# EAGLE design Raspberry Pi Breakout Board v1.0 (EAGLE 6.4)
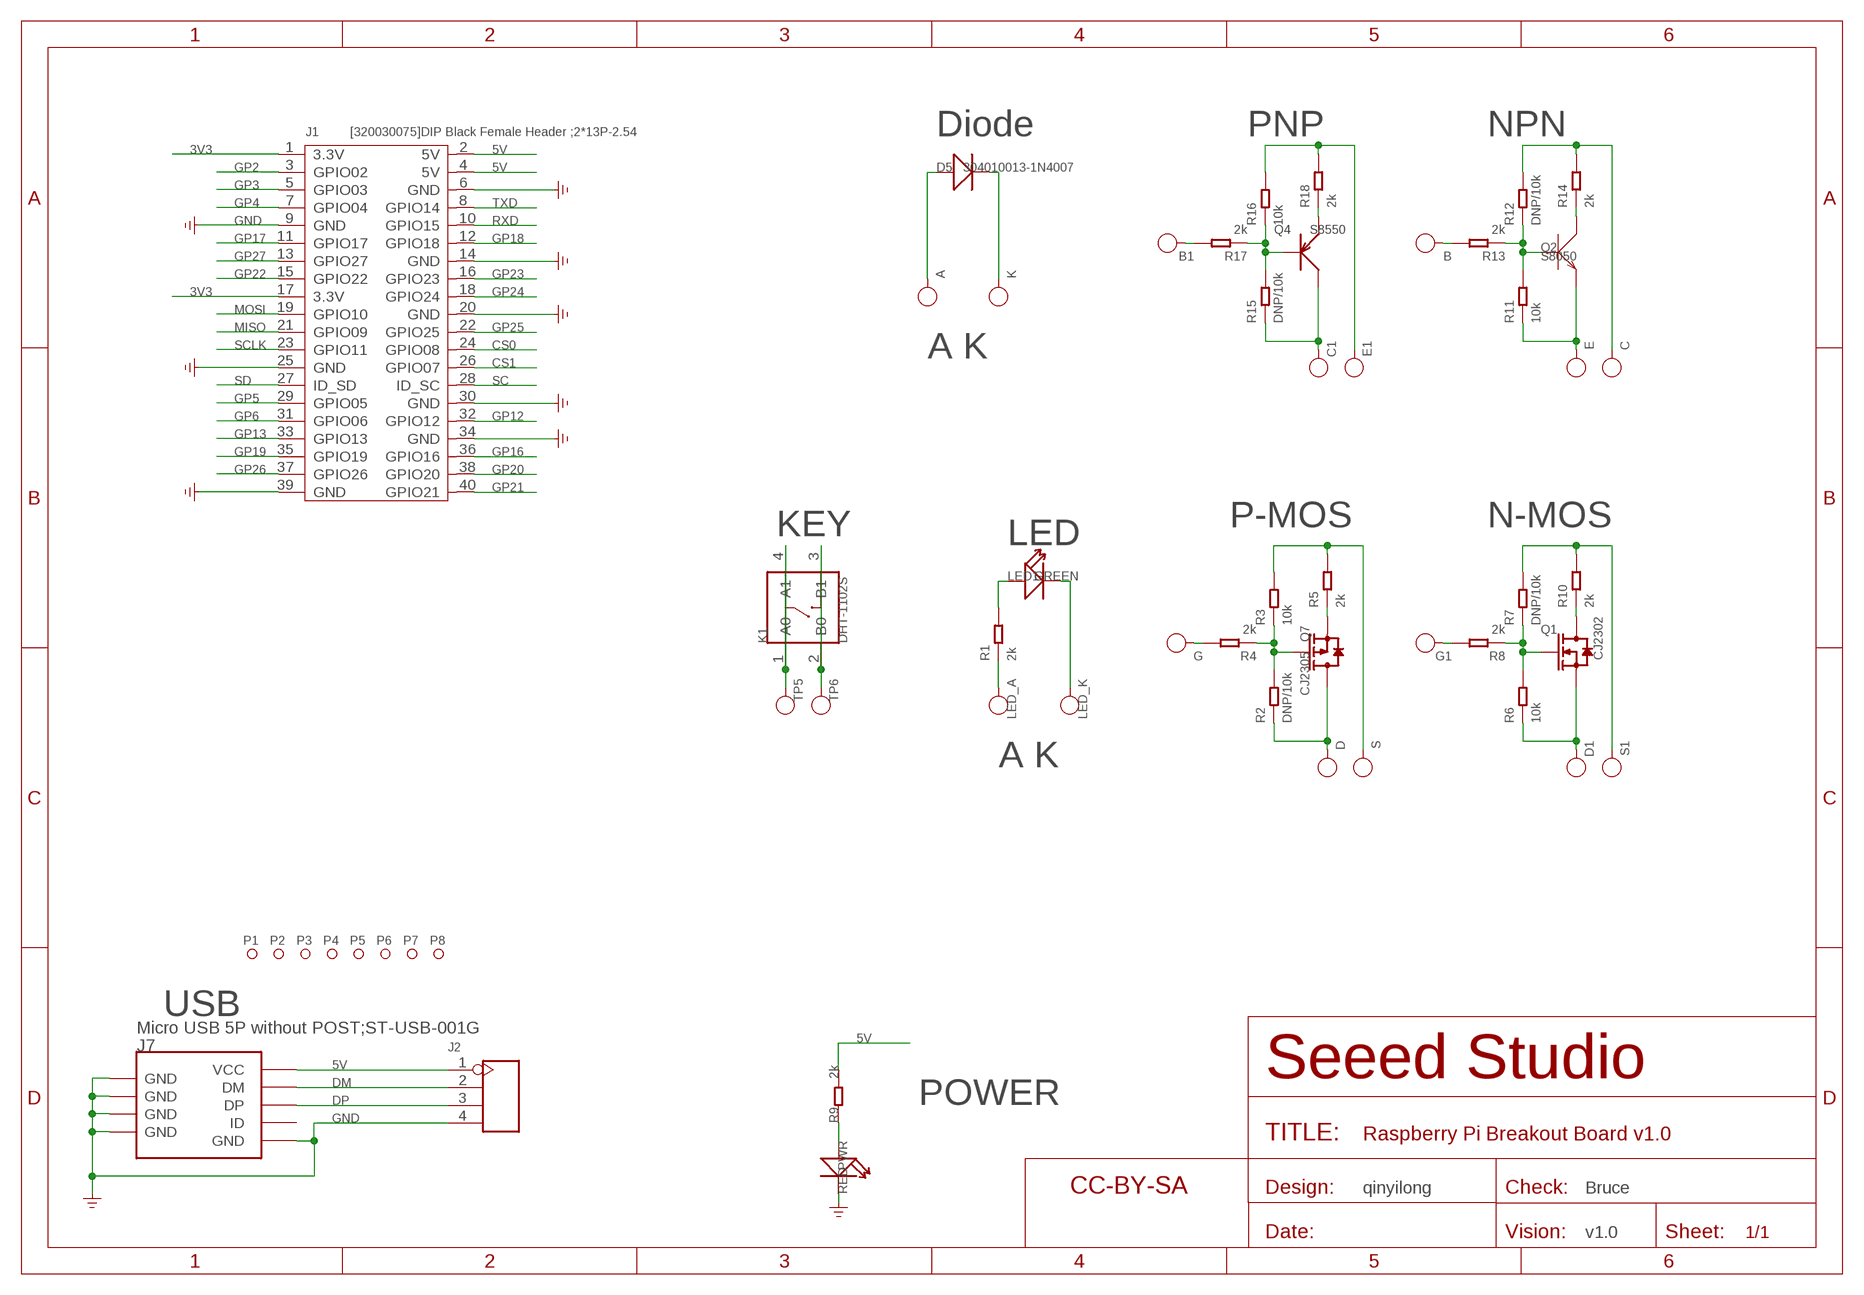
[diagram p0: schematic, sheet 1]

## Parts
A  PAD-TEST-POINT'4080'  [PAD-L80*W40MIL]
B  PAD-TEST-POINT'4080'  [PAD-L80*W40MIL]
B1  PAD-TEST-POINT'4080'  [PAD-L80*W40MIL]
C  PAD-TEST-POINT'4080'  [PAD-L80*W40MIL]
C1  PAD-TEST-POINT'4080'  [PAD-L80*W40MIL]
D  PAD-TEST-POINT'4080'  [PAD-L80*W40MIL]
D1  PAD-TEST-POINT'4080'  [PAD-L80*W40MIL]
D5  304010013-1N4007  D'DO-214AC'  [D2010]
E  PAD-TEST-POINT'4080'  [PAD-L80*W40MIL]
E1  PAD-TEST-POINT'4080'  [PAD-L80*W40MIL]
G  PAD-TEST-POINT'4080'  [PAD-L80*W40MIL]
G1  PAD-TEST-POINT'4080'  [PAD-L80*W40MIL]
J1  [320030075]DIP Black Female Header ;2*13P-2.54  HEADER-2X20P  [2X20P-2.54-65/35MIL]
J2  HEADER-4P-65/35MIL  [4P-2.54-65/35MIL]
J7  Micro USB 5P without POST;ST-USB-001G  USB-MINIUSB-5P-MICRO  [MICRO-USB]
K  PAD-TEST-POINT'4080'  [PAD-L80*W40MIL]
K1  DHT-1102S  BUTTON-4PDTSM-62K-S-V-T/R(SN431)  [4P-SMD-L6.0*W6.0*H5.0MM]
LED1  GREEN  LED'0603'  [LED-0603]
LED_A  PAD-TEST-POINT'4080'  [PAD-L80*W40MIL]
LED_K  PAD-TEST-POINT'4080'  [PAD-L80*W40MIL]
P1  PAD-MARK'ANNULAR'  [ROUND-MARK-1.0]
P2  PAD-MARK'ANNULAR'  [ROUND-MARK-1.0]
P3  PAD-MARK'ANNULAR'  [ROUND-MARK-1.0]
P4  PAD-MARK'ANNULAR'  [ROUND-MARK-1.0]
P5  PAD-MARK'ANNULAR'  [ROUND-MARK-1.0]
P6  PAD-MARK'ANNULAR'  [ROUND-MARK-1.0]
P7  PAD-MARK'ANNULAR'  [ROUND-MARK-1.0]
P8  PAD-MARK'ANNULAR'  [ROUND-MARK-1.0]
PWR  RED  LED'0603'  [LED-0603]
Q1  CJ2302  MOSFET-N'SOT23'  [SOT23]
Q2  S8050  TRANSISTOR-NPN-SOT23  [SOT23]
Q4  S8550  TRANSISTOR-PNP-SOT23  [SOT23]
Q7  CJ2305  MOSFET-P'SI2323CDS/SI2305DS<BR>'  [SOT23]
R1  2k  RES-0603  [R0603]
R2  DNP/10k  RES-0603  [R0603]
R3  10k  RES-0603  [R0603]
R4  2k  RES-0603  [R0603]
R5  2k  RES-0603  [R0603]
R6  10k  RES-0603  [R0603]
R7  DNP/10k  RES-0603  [R0603]
R8  2k  RES-0603  [R0603]
R9  2k  R-0603  [R0603]
R10  2k  RES-0603  [R0603]
R11  10k  RES-0603  [R0603]
R12  DNP/10k  RES-0603  [R0603]
R13  2k  RES-0603  [R0603]
R14  2k  RES-0603  [R0603]
R15  DNP/10k  RES-0603  [R0603]
R16  10k  RES-0603  [R0603]
R17  2k  RES-0603  [R0603]
R18  2k  RES-0603  [R0603]
S  PAD-TEST-POINT'4080'  [PAD-L80*W40MIL]
S1  PAD-TEST-POINT'4080'  [PAD-L80*W40MIL]
TP5  PAD-TEST-POINT'4080'  [PAD-L80*W40MIL]
TP6  PAD-TEST-POINT'4080'  [PAD-L80*W40MIL]
U$2  SEEEDSTUDIO-OPEN-SCH-FRAME  [SEEEDSTUDIO-PCB-FRAME]

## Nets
3V3: J1.1(3.3V) J1.17(3.3V)
5V: J1.2(5V) J1.4(5V) J2.1 J7.1(VCC) R9.2
CS0: J1.24(GPIO08)
CS1: J1.26(GPIO07)
DM: J2.2 J7.2(DM)
DP: J2.3 J7.3(DP)
GND: J1.6(GND) J1.9(GND) J1.14(GND) J1.20(GND) J1.25(GND) J1.30(GND) J1.34(GND) J1.39(GND) J2.4 J7.5(GND) J7.S1(GND) J7.S2(GND) J7.S3(GND) J7.S4(GND) J7.S5(GND) J7.S6(GND) PWR.- ; supply symbol labelled GND_POWER
GP2: J1.3(GPIO02)
GP3: J1.5(GPIO03)
GP4: J1.7(GPIO04)
GP5: J1.29(GPIO05)
GP6: J1.31(GPIO06)
GP12: J1.32(GPIO12)
GP13: J1.33(GPIO13)
GP16: J1.36(GPIO16)
GP17: J1.11(GPIO17)
GP18: J1.12(GPIO18)
GP19: J1.35(GPIO19)
GP20: J1.38(GPIO20)
GP21: J1.40(GPIO21)
GP22: J1.15(GPIO22)
GP23: J1.16(GPIO23)
GP24: J1.18(GPIO24)
GP25: J1.22(GPIO25)
GP26: J1.37(GPIO26)
GP27: J1.13(GPIO27)
MISO: J1.21(GPIO09)
MOSI: J1.19(GPIO10)
N$320: LED_A.1(T) R1.1
N$336: C1.1(T) Q4.3(C) R15.1
N$347: Q7.1(G) R2.2 R3.1 R4.1
N$370: R3.2 R5.2 S.1(T)
N$373: D1.1(T) Q1.2(S) R6.1
N$374: G.1(T) R4.2
N$375: Q7.2(S) R5.1
N$376: Q1.1(G) R6.2 R7.1 R8.1
N$377: PWR.+ R9.1
N$378: Q4.1(B) R15.2 R16.1 R17.1
N$379: E1.1(T) R16.2 R18.2
N$380: B1.1(T) R17.2
N$381: Q4.2(E) R18.1
N$383: R7.2 R10.2 S1.1(T)
N$384: G1.1(T) R8.2
N$385: D.1(T) Q7.3(D) R2.1
N$386: E.1(T) Q2.2(E) R11.1
N$387: Q2.1(B) R11.2 R12.1 R13.1
N$388: C.1(T) R12.2 R14.2
N$389: A.1(T) D5.+
N$390: D5.- K.1(T)
N$391: LED1.+ R1.2
N$392: LED1.- LED_K.1(T)
N$393: K1.1(A0) K1.4(A1) TP5.1(T)
N$394: K1.2(B0) K1.3(B1) TP6.1(T)
N$395: Q1.3(D) R10.1
N$396: B.1(T) R13.2
N$397: Q2.3(C) R14.1
RXD: J1.10(GPIO15)
SC: J1.28(ID_SC)
SCLK: J1.23(GPIO11)
SD: J1.27(ID_SD)
TXD: J1.8(GPIO14)
Unconnected: J7.4(ID)

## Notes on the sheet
- Diode | PNP | NPN
- A K
- KEY | P-MOS | N-MOS
- LED
- A K
- USB
- POWER
- qinyilong | Bruce
- v1.0

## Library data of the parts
A B B1 C C1 D D1 E E1 G G1 K LED_A LED_K S S1 TP5 TP6 = Discrete-new:PAD-TEST-POINT
D5 = Discrete:D*
J1 = Connector-new:HEADER-2X20P
J2 = Connector-new:HEADER-4P
J7 = Connector :USB-MINIUSB-5P
K1 = Discrete-new:BUTTON-4P: 4P-L6.0*W6.0*H5.0mm:311020024;4P-L8.0*W8.0*H9.0MM:311020028;4P-SMD-L6.0*W6.0*H5.0MM:311020004;4P-SMD-L3.35*W3.35*H1.5MM:311020030;4P-SMD-L5.2*W5.2*H2.5:311020046
LED1 PWR = Discrete:LED*
P1-P8 = Discrete-new:PAD-MARK; PARTNO: DNP
Q1 = Discrete:MOSFET-N: IRLL014: http://www.vishay.com/docs/91319/sihll014.pdf
Q2 = Discrete:TRANSISTOR-NPN*: NPN audion
Q4 = Discrete:TRANSISTOR-PNP*: PNP audion
Q7 = Discrete:MOSFET-P
R1-R8 R10-R18 = Discrete-new:RES
R9 = Discrete:R*
U$2 = moudle-new:SEEEDSTUDIO-OPEN-SCH-FRAME

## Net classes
0 default: width 0.076 mm, drill 0.102 mm, clearance 0.076 mm

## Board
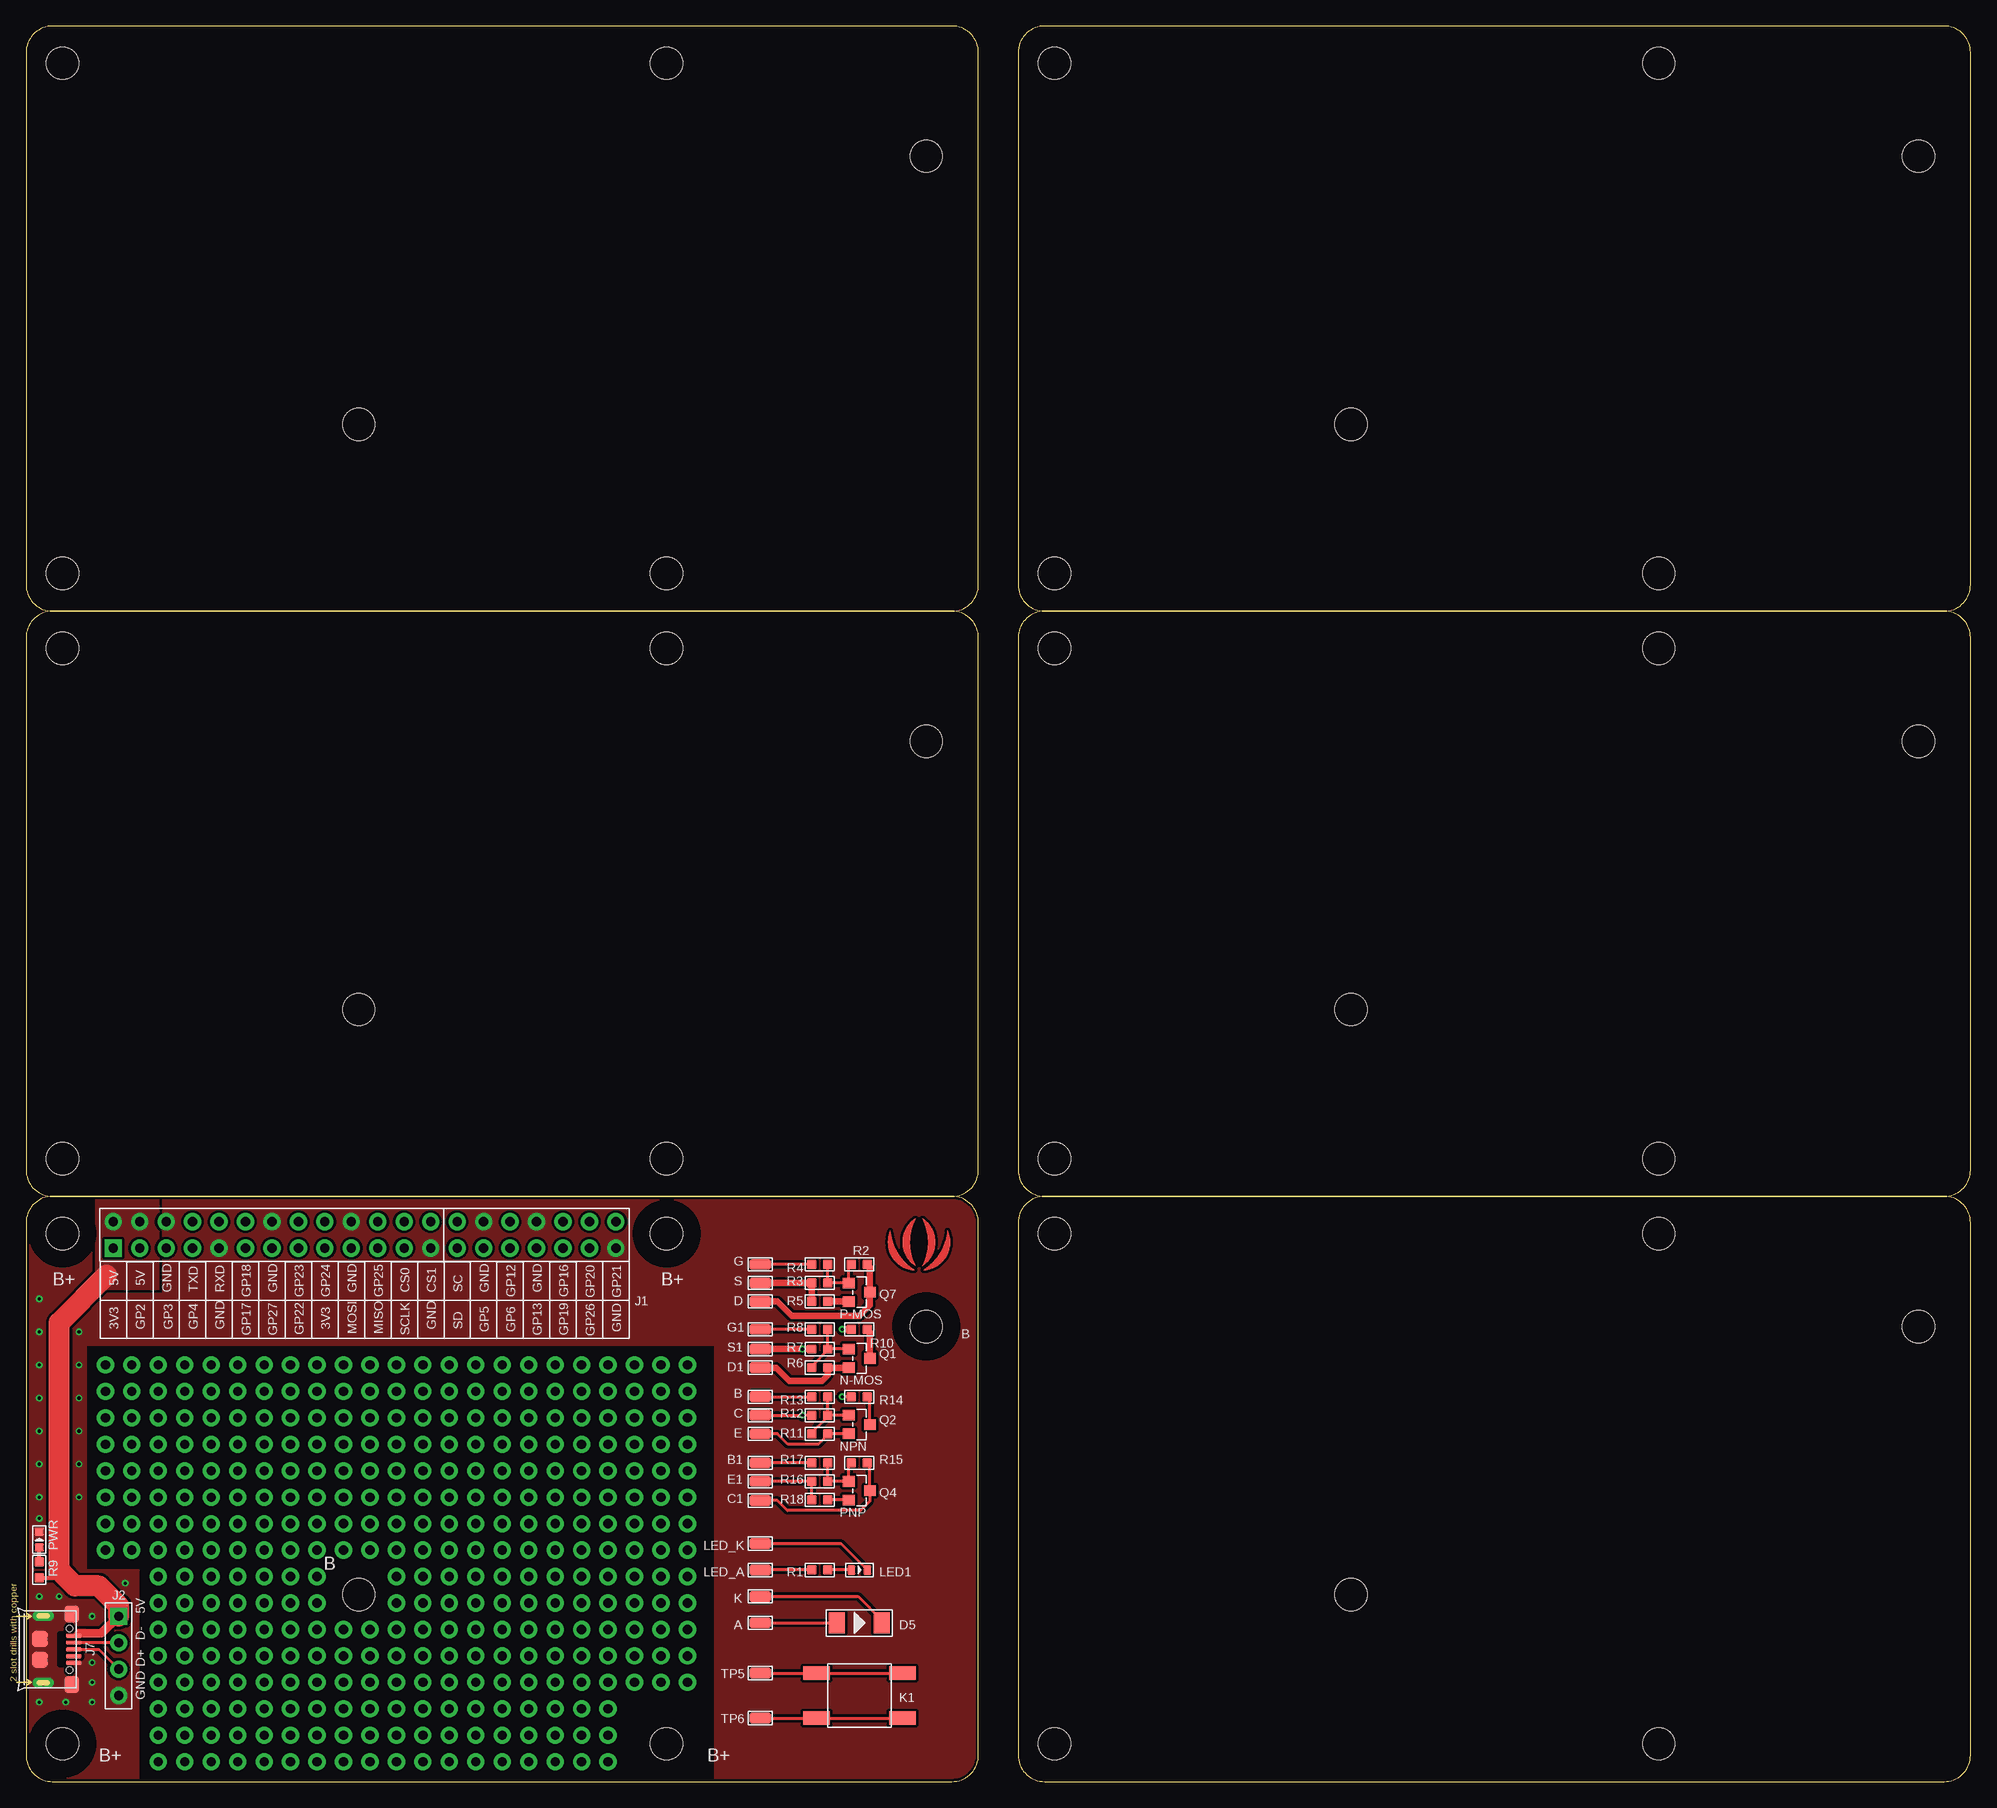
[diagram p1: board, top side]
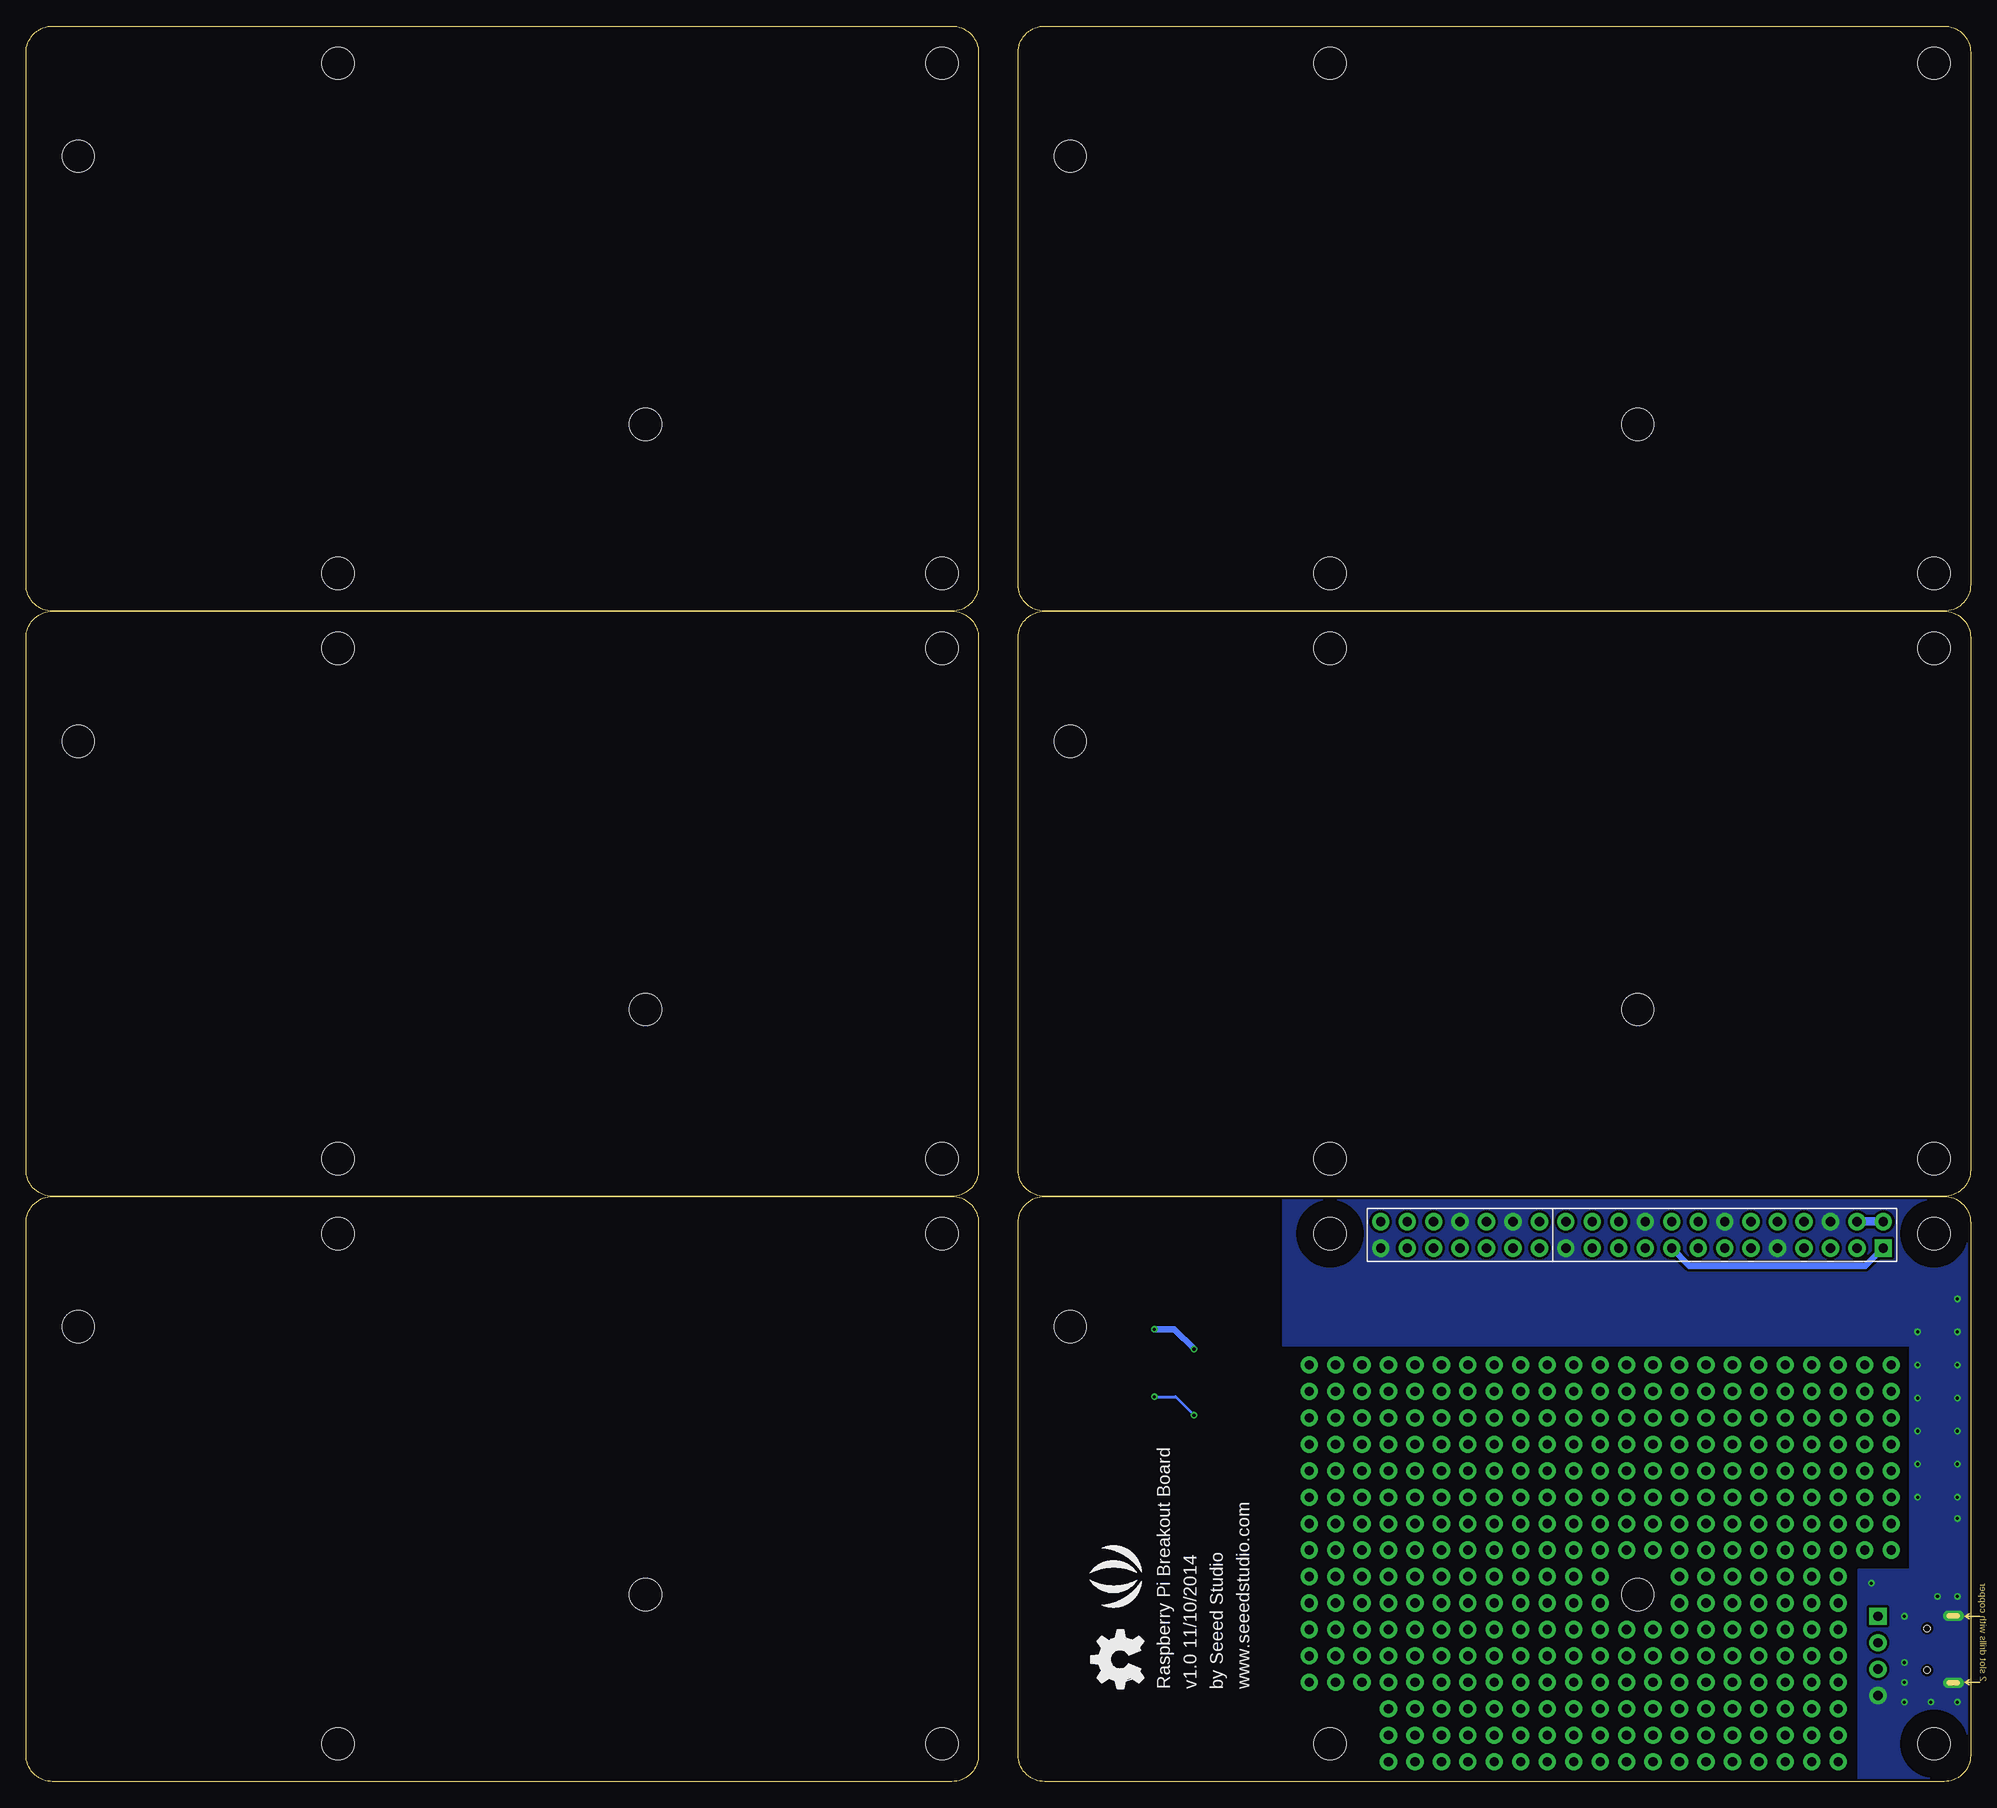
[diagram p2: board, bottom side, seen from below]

Size 186.69 x 168.59 mm. Coordinates in mm from the lower left corner, seen from the top.
Copper layers (1*16): Top 0.035mm / dielectric 1.5mm / Bottom 0.035mm
Design rules "SeeedStudio_2layer_DRU_no_angle_20140221 *": minimum track width 6mil, minimum drill 12mil, track to track 6mil, track to pad 6mil, pad to pad 6mil, via to via 6mil, smd to smd 0mil, copper to edge 10mil, drill to drill 10mil, minimum pad ring 10mil, minimum via ring 6mil, stop-mask expansion 2mil, vias tented up to drill 25mil, thermal gap 10mil
Holes 2.03 mm at 183.01,173.74 2.79,-4.19 2.79,173.74 183.01,-5.08

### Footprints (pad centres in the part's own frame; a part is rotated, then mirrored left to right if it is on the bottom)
PAD-L80*W40MIL = smd 2.032 x 1.016: 1 0,0
D2010 = smd 1.524 x 2.032: + -2.159,0; - 2.159,0
2X20P-2.54-65/35MIL = drill 0.889 pad 1.651 square: 1 1.27,24.13 | drill 0.889 pad 1.651: 2 -1.27,24.13; 3 1.27,21.59; 4 -1.27,21.59; 5 1.27,19.05; 6 -1.27,19.05; 7 1.27,16.51; 8 -1.27,16.51; 9 1.27,13.97; 10 -1.27,13.97; 11 1.27,11.43; 12 -1.27,11.43; 13 1.27,8.89; 14 -1.27,8.89; 15 1.27,6.35; 16 -1.27,6.35; 17 1.27,3.81; 18 -1.27,3.81; 19 1.27,1.27; 20 -1.27,1.27; 21 1.27,-1.27; 22 -1.27,-1.27; 23 1.27,-3.81; 24 -1.27,-3.81; 25 1.27,-6.35; 26 -1.27,-6.35; 27 1.27,-8.89; 28 -1.27,-8.89; 29 1.27,-11.43; 30 -1.27,-11.43; 31 1.27,-13.97; 32 -1.27,-13.97; 33 1.27,-16.51; 34 -1.27,-16.51; 35 1.27,-19.05; 36 -1.27,-19.05; 37 1.27,-21.59; 38 -1.27,-21.59; 39 1.27,-24.13; 40 -1.27,-24.13
4P-2.54-65/35MIL = drill 0.889 pad 1.651 square: 1 0,3.81 | drill 0.889 pad 1.651: 2 0,1.27; 3 0,-1.27; 4 0,-3.81
MICRO-USB = smd 0.381 x 1.524: 1 -1.3,-0.25; 2 -0.65,-0.25; 3 0,-0.25; 4 0.65,-0.25; 5 1.3,-0.25 | smd 1.6 x 1.397: S1 -3.4,-0.427; S6 3.4,-0.427 | drill 0.508 pad 1.016 long: S2 -3.226,-3.175; S5 3.226,-3.175 | smd 1.5 x 1.5: S3 -1,-3.5; S4 1,-3.5 | hole 0.635: -2,-0.65; 2,-0.65
4P-SMD-L6.0*W6.0*H5.0MM = smd 2.54 x 1.27: 1 -4.129,2.159; 2 -4.129,-2.159; 3 4.129,-2.159; 4 4.129,2.159
LED-0603 = smd 0.762 x 0.889: + -0.762,0; - 0.762,0
ROUND-MARK-1.0 = smd 1.016 x 1.016: P$1 0,0
SOT23 = smd 1.016 x 1.143: 1 -0.889,-1.016; 2 0.889,-1.016; 3 0,1.016
R0603 = smd 0.889 x 0.889: 1 -0.762,0; 2 0.762,0
RASPBERRY-PI-B+/B = hole 3.1: 3.503,52.622; 3.503,3.622; 61.503,52.622; 61.503,3.622; 31.951,17.951; 86.431,43.7

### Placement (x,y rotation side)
A  70.48,15.24 180 top
B  70.48,36.96 180 top
B1  70.48,30.61 180 top
C  70.48,35.18 180 top
C1  70.48,26.99 0 top
D  70.48,46.1 180 top
D1  70.48,39.75 180 top
D5  80.01,15.24 0 top
E  70.48,33.4 180 top
E1  70.48,28.83 180 top
G  70.48,49.66 180 top
G1  70.48,43.43 180 top
J1  32.5,52.5 270 bottom
J2  8.89,12.06 0 top
J7  4.83,12.7 270 top
K  70.48,17.78 180 top
K1  80.01,8.26 0 top
LED1  80.01,20.32 0 top
LED_A  70.48,20.32 0 top
LED_K  70.48,22.86 0 top
P1  not placed on the board
P2  not placed on the board
P3  not placed on the board
P4  not placed on the board
P5  not placed on the board
P6  not placed on the board
P7  not placed on the board
P8  not placed on the board
PWR  1.27,23.24 90 top
Q1  80.01,40.64 270 top
Q2  80.01,34.29 270 top
Q4  80.01,27.94 270 top
Q7  80.01,46.99 270 top
R1  76.2,20.32 0 top
R2  80.01,49.66 180 top
R3  76.2,47.88 180 top
R4  76.2,49.66 180 top
R5  76.2,46.1 180 top
R6  76.2,39.75 180 top
R7  76.2,41.53 180 top
R8  76.2,43.43 180 top
R9  1.27,20.32 270 top
R10  80.01,43.43 180 top
R11  76.2,33.4 180 top
R12  76.2,35.18 180 top
R13  76.2,36.96 180 top
R14  80.01,36.96 180 top
R15  80.01,30.61 180 top
R16  76.2,28.83 180 top
R17  76.2,30.61 180 top
R18  76.2,27.05 180 top
S  70.48,47.88 0 top
S1  70.48,41.53 0 top
TP5  70.48,10.41 0 top
TP6  70.48,6.1 0 top
U$1  [RASPBERRY-PI-B+/B]  95.25,0 0 top
U$2  not placed on the board
U$3  [RASPBERRY-PI-B+/B]  0,0 0 top
U$5  [RASPBERRY-PI-B+/B]  95.25,112.39 0 top
U$6  [SEEED-COPPER-280*268MIL]  85.72,50.8 0 top
U$7  [RASPBERRY-PI-B+/B]  0,56.2 0 top
U$8  [RASPBERRY-PI-B+/B]  0,112.39 0 top
U$12  [OSHW_FILLX200_NOTEXT]  79.38,8.89 90 bottom
U$17  [SEEED-SILK-280*268MIL]  81.28,19.68 90 bottom
U$18  [RASPBERRY-PI-B+/B]  95.25,56.2 0 top

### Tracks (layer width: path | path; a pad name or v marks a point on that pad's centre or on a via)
3V3
  Bottom 0.61: J1.1 8.4,51.23 10.1,49.53 26.99,49.53 J1.17
5V
  Top 0.406: R9.2 2.16,19.56 | 2.16,19.56 2.41,19.56 | 2.41,19.56 3.17,19.56 3.3,19.68 3.81,19.68 | 2.41,19.56 2.41,19.81 | 2.41,19.81 2.41,20.32 | 2.41,19.81 2.16,19.56
  Top 0.813: 5.08,14.22 7.24,14.22 J2.1
  Top 2.032: J2.1 8.89,16.89 6.99,18.8 4.7,18.8 3.81,19.68 3.17,20.32 3.17,44.07 7.75,48.64
  Bottom 0.813: J1.4 J1.2
  pour Top (isolate 0.254, no thermals): 6.73,56.01 12.7,56.01 12.7,47.24 6.73,47.24
  pour Top (isolate 0.254, no thermals): 3.81,13.91 3.81,14.61 5.71,14.61 5.71,13.91
DM
  Top 0.305: J7.2 8.88,13.35 J2.2
DP
  Top 0.305: J7.3 6.99,12.7 J2.3
GND  (via drill 0.3 pad 0.64)
  other vias: 6.35,11.43 6.35,9.53 6.35,7.62 6.35,15.88 9.53,19.05 3.17,17.78 3.81,7.62 1.27,7.62 1.27,25.27 1.27,27.3 1.27,30.48 1.27,33.66 1.27,36.83 1.27,40.01 1.27,43.18 1.27,46.35 5.08,27.3 5.08,30.48 5.08,33.66 5.08,36.83 5.08,40.01 5.08,43.18 1.27,17.78
  pour Bottom (isolate 0.254, rank 6, no thermals): -0.64,56.52 66.04,56.52 66.04,41.91 5.84,41.91 5.84,20.32 10.79,20.32 10.79,-0.64 -0.64,-0.64
  pour Top (isolate 0.254, rank 6, no thermals): -0.64,56.52 92.08,56.52 92.08,-0.64 66.17,-0.64 66.17,41.91 5.71,41.91 5.71,20.32 10.79,20.32 10.79,-0.64 -0.64,-0.64
N$1  (via drill 0.89 pad 1.65)
  other vias: 10.16,27.3
N$2  (via drill 0.89 pad 1.65)
  other vias: 38.1,32.38
N$3  (via drill 0.89 pad 1.65)
  other vias: 12.7,27.3
N$4  (via drill 0.89 pad 1.65)
  other vias: 40.64,32.38
N$5  (via drill 0.89 pad 1.65)
  other vias: 15.24,27.3
N$6  (via drill 0.89 pad 1.65)
  other vias: 17.78,27.3
N$7  (via drill 0.89 pad 1.65)
  other vias: 20.32,27.3
N$8  (via drill 0.89 pad 1.65)
  other vias: 22.86,27.3
N$9  (via drill 0.89 pad 1.65)
  other vias: 25.4,27.3
N$10  (via drill 0.89 pad 1.65)
  other vias: 27.94,27.3
N$11  (via drill 0.89 pad 1.65)
  other vias: 30.48,27.3
N$12  (via drill 0.89 pad 1.65)
  other vias: 38.1,24.77
N$13  (via drill 0.89 pad 1.65)
  other vias: 38.1,22.23
N$14  (via drill 0.89 pad 1.65)
  other vias: 33.02,27.3
N$15  (via drill 0.89 pad 1.65)
  other vias: 38.1,19.68
N$16  (via drill 0.89 pad 1.65)
  other vias: 40.64,24.77
N$17  (via drill 0.89 pad 1.65)
  other vias: 40.64,22.23
N$18  (via drill 0.89 pad 1.65)
  other vias: 40.64,19.68
N$19  (via drill 0.89 pad 1.65)
  other vias: 43.18,24.77
N$20  (via drill 0.89 pad 1.65)
  other vias: 43.18,22.23
N$21  (via drill 0.89 pad 1.65)
  other vias: 43.18,19.68
N$22  (via drill 0.89 pad 1.65)
  other vias: 45.72,24.77
N$23  (via drill 0.89 pad 1.65)
  other vias: 45.72,22.23
N$24  (via drill 0.89 pad 1.65)
  other vias: 45.72,19.68
N$25  (via drill 0.89 pad 1.65)
  other vias: 48.26,24.77
N$26  (via drill 0.89 pad 1.65)
  other vias: 48.26,22.23
N$27  (via drill 0.89 pad 1.65)
  other vias: 48.26,19.68
N$28  (via drill 0.89 pad 1.65)
  other vias: 50.8,24.77
N$29  (via drill 0.89 pad 1.65)
  other vias: 50.8,22.23
N$30  (via drill 0.89 pad 1.65)
  other vias: 50.8,19.68
N$31  (via drill 0.89 pad 1.65)
  other vias: 53.34,24.77
N$32  (via drill 0.89 pad 1.65)
  other vias: 53.34,22.23
N$33  (via drill 0.89 pad 1.65)
  other vias: 53.34,19.68
N$34  (via drill 0.89 pad 1.65)
  other vias: 55.88,24.77
N$35  (via drill 0.89 pad 1.65)
  other vias: 55.88,22.23
N$36  (via drill 0.89 pad 1.65)
  other vias: 55.88,19.68
N$37  (via drill 0.89 pad 1.65)
  other vias: 58.42,24.77
N$38  (via drill 0.89 pad 1.65)
  other vias: 58.42,22.23
N$39  (via drill 0.89 pad 1.65)
  other vias: 58.42,19.68
N$40  (via drill 0.89 pad 1.65)
  other vias: 60.96,24.77
N$41  (via drill 0.89 pad 1.65)
  other vias: 60.96,22.23
N$42  (via drill 0.89 pad 1.65)
  other vias: 60.96,19.68
N$43  (via drill 0.89 pad 1.65)
  other vias: 43.18,32.38
N$44  (via drill 0.89 pad 1.65)
  other vias: 45.72,32.38
N$45  (via drill 0.89 pad 1.65)
  other vias: 48.26,32.38
N$46  (via drill 0.89 pad 1.65)
  other vias: 10.16,24.77
N$47  (via drill 0.89 pad 1.65)
  other vias: 38.1,12.06
N$48  (via drill 0.89 pad 1.65)
  other vias: 50.8,32.38
N$49  (via drill 0.89 pad 1.65)
  other vias: 12.7,24.77
N$50  (via drill 0.89 pad 1.65)
  other vias: 10.16,34.92
N$51  (via drill 0.89 pad 1.65)
  other vias: 15.24,24.77
N$52  (via drill 0.89 pad 1.65)
  other vias: 38.1,9.53
N$53  (via drill 0.89 pad 1.65)
  other vias: 53.34,32.38
N$54  (via drill 0.89 pad 1.65)
  other vias: 38.1,17.14
N$55  (via drill 0.89 pad 1.65)
  other vias: 38.1,27.3
N$56  (via drill 0.89 pad 1.65)
  other vias: 38.1,14.61
N$58  (via drill 0.89 pad 1.65)
  other vias: 40.64,17.14
N$59  (via drill 0.89 pad 1.65)
  other vias: 40.64,14.61
N$60  (via drill 0.89 pad 1.65)
  other vias: 40.64,12.06
N$61  (via drill 0.89 pad 1.65)
  other vias: 43.18,17.14
N$62  (via drill 0.89 pad 1.65)
  other vias: 43.18,14.61
N$63  (via drill 0.89 pad 1.65)
  other vias: 40.64,9.53
N$64  (via drill 0.89 pad 1.65)
  other vias: 45.72,17.14
N$65  (via drill 0.89 pad 1.65)
  other vias: 45.72,14.61
N$67  (via drill 0.89 pad 1.65)
  other vias: 48.26,17.14
N$68  (via drill 0.89 pad 1.65)
  other vias: 48.26,14.61
N$69  (via drill 0.89 pad 1.65)
  other vias: 43.18,12.06
N$70  (via drill 0.89 pad 1.65)
  other vias: 50.8,17.14
N$71  (via drill 0.89 pad 1.65)
  other vias: 50.8,14.61
N$72  (via drill 0.89 pad 1.65)
  other vias: 43.18,9.53
N$73  (via drill 0.89 pad 1.65)
  other vias: 53.34,17.14
N$74  (via drill 0.89 pad 1.65)
  other vias: 53.34,14.61
N$75  (via drill 0.89 pad 1.65)
  other vias: 45.72,12.06
N$76  (via drill 0.89 pad 1.65)
  other vias: 55.88,17.14
N$77  (via drill 0.89 pad 1.65)
  other vias: 55.88,14.61
N$79  (via drill 0.89 pad 1.65)
  other vias: 58.42,17.14
N$80  (via drill 0.89 pad 1.65)
  other vias: 58.42,14.61
N$81  (via drill 0.89 pad 1.65)
  other vias: 45.72,9.53
N$82  (via drill 0.89 pad 1.65)
  other vias: 60.96,17.14
N$83  (via drill 0.89 pad 1.65)
  other vias: 60.96,14.61
N$85  (via drill 0.89 pad 1.65)
  other vias: 55.88,32.38
N$86  (via drill 0.89 pad 1.65)
  other vias: 58.42,32.38
N$87  (via drill 0.89 pad 1.65)
  other vias: 60.96,32.38
N$88  (via drill 0.89 pad 1.65)
  other vias: 48.26,12.06
N$89  (via drill 0.89 pad 1.65)
  other vias: 48.26,9.53
N$90  (via drill 0.89 pad 1.65)
  other vias: 50.8,12.06
N$91  (via drill 0.89 pad 1.65)
  other vias: 50.8,9.53
N$92  (via drill 0.89 pad 1.65)
  other vias: 53.34,12.06
N$93  (via drill 0.89 pad 1.65)
  other vias: 53.34,9.53
N$94  (via drill 0.89 pad 1.65)
  other vias: 55.88,12.06
N$95  (via drill 0.89 pad 1.65)
  other vias: 55.88,9.53
N$96  (via drill 0.89 pad 1.65)
  other vias: 58.42,12.06
N$97  (via drill 0.89 pad 1.65)
  other vias: 58.42,9.53
N$98  (via drill 0.89 pad 1.65)
  other vias: 60.96,12.06
N$99  (via drill 0.89 pad 1.65)
  other vias: 40.64,27.3
N$101  (via drill 0.89 pad 1.65)
  other vias: 60.96,9.53
N$102  (via drill 0.89 pad 1.65)
  other vias: 30.48,6.99
N$103  (via drill 0.89 pad 1.65)
  other vias: 30.48,4.45
N$104  (via drill 0.89 pad 1.65)
  other vias: 33.02,6.99
N$105  (via drill 0.89 pad 1.65)
  other vias: 33.02,4.45
N$106  (via drill 0.89 pad 1.65)
  other vias: 35.56,6.99
N$107  (via drill 0.89 pad 1.65)
  other vias: 35.56,4.45
N$108  (via drill 0.89 pad 1.65)
  other vias: 17.78,24.77
N$109  (via drill 0.89 pad 1.65)
  other vias: 38.1,6.99
N$110  (via drill 0.89 pad 1.65)
  other vias: 40.64,34.92
N$111  (via drill 0.89 pad 1.65)
  other vias: 43.18,34.92
N$112  (via drill 0.89 pad 1.65)
  other vias: 38.1,4.45
N$113  (via drill 0.89 pad 1.65)
  other vias: 45.72,34.92
N$114  (via drill 0.89 pad 1.65)
  other vias: 48.26,34.92
N$115  (via drill 0.89 pad 1.65)
  other vias: 40.64,6.99
N$116  (via drill 0.89 pad 1.65)
  other vias: 50.8,34.92
N$117  (via drill 0.89 pad 1.65)
  other vias: 53.34,34.92
N$119  (via drill 0.89 pad 1.65)
  other vias: 55.88,34.92
N$120  (via drill 0.89 pad 1.65)
  other vias: 58.42,34.92
N$122  (via drill 0.89 pad 1.65)
  other vias: 60.96,34.92
N$124  (via drill 0.89 pad 1.65)
  other vias: 40.64,4.45
N$125  (via drill 0.89 pad 1.65)
  other vias: 43.18,6.99
N$126  (via drill 0.89 pad 1.65)
  other vias: 43.18,4.45
N$127  (via drill 0.89 pad 1.65)
  other vias: 45.72,6.99
N$128  (via drill 0.89 pad 1.65)
  other vias: 45.72,4.45
N$129  (via drill 0.89 pad 1.65)
  other vias: 48.26,6.99
N$130  (via drill 0.89 pad 1.65)
  other vias: 48.26,4.45
N$131  (via drill 0.89 pad 1.65)
  other vias: 50.8,6.99
N$132  (via drill 0.89 pad 1.65)
  other vias: 50.8,4.45
N$133  (via drill 0.89 pad 1.65)
  other vias: 63.5,34.92
N$134  (via drill 0.89 pad 1.65)
  other vias: 63.5,32.38
N$135  (via drill 0.89 pad 1.65)
  other vias: 63.5,29.84
N$136  (via drill 0.89 pad 1.65)
  other vias: 63.5,27.3
N$137  (via drill 0.89 pad 1.65)
  other vias: 63.5,24.77
N$138  (via drill 0.89 pad 1.65)
  other vias: 63.5,22.23
N$139  (via drill 0.89 pad 1.65)
  other vias: 63.5,19.68
N$141  (via drill 0.89 pad 1.65)
  other vias: 63.5,17.14
N$142  (via drill 0.89 pad 1.65)
  other vias: 63.5,14.61
N$143  (via drill 0.89 pad 1.65)
  other vias: 43.18,27.3
N$144  (via drill 0.89 pad 1.65)
  other vias: 53.34,6.99
N$145  (via drill 0.89 pad 1.65)
  other vias: 53.34,4.45
N$146  (via drill 0.89 pad 1.65)
  other vias: 35.56,22.23
N$147  (via drill 0.89 pad 1.65)
  other vias: 20.32,24.77
N$148  (via drill 0.89 pad 1.65)
  other vias: 7.62,27.3
N$156  (via drill 0.89 pad 1.65)
  other vias: 38.1,29.84
N$157  (via drill 0.89 pad 1.65)
  other vias: 40.64,29.84
N$158  (via drill 0.89 pad 1.65)
  other vias: 43.18,29.84
N$159  (via drill 0.89 pad 1.65)
  other vias: 45.72,29.84
N$160  (via drill 0.89 pad 1.65)
  other vias: 48.26,29.84
N$161  (via drill 0.89 pad 1.65)
  other vias: 50.8,29.84
N$162  (via drill 0.89 pad 1.65)
  other vias: 53.34,29.84
N$163  (via drill 0.89 pad 1.65)
  other vias: 55.88,29.84
N$164  (via drill 0.89 pad 1.65)
  other vias: 58.42,29.84
N$165  (via drill 0.89 pad 1.65)
  other vias: 60.96,29.84
N$166  (via drill 0.89 pad 1.65)
  other vias: 22.86,24.77
N$167  (via drill 0.89 pad 1.65)
  other vias: 63.5,12.06
N$168  (via drill 0.89 pad 1.65)
  other vias: 25.4,24.77
N$169  (via drill 0.89 pad 1.65)
  other vias: 10.16,40.01
N$170  (via drill 0.89 pad 1.65)
  other vias: 27.94,24.77
N$171  (via drill 0.89 pad 1.65)
  other vias: 35.56,19.68
N$172  (via drill 0.89 pad 1.65)
  other vias: 30.48,24.77
N$173  (via drill 0.89 pad 1.65)
  other vias: 38.1,40.01
N$174  (via drill 0.89 pad 1.65)
  other vias: 33.02,24.77
N$175  (via drill 0.89 pad 1.65)
  other vias: 10.16,22.23
N$176  (via drill 0.89 pad 1.65)
  other vias: 10.16,29.84
N$177  (via drill 0.89 pad 1.65)
  other vias: 12.7,29.84
N$178  (via drill 0.89 pad 1.65)
  other vias: 15.24,29.84
N$179  (via drill 0.89 pad 1.65)
  other vias: 17.78,29.84
N$180  (via drill 0.89 pad 1.65)
  other vias: 20.32,29.84
N$181  (via drill 0.89 pad 1.65)
  other vias: 22.86,29.84
N$182  (via drill 0.89 pad 1.65)
  other vias: 63.5,9.53
N$185  (via drill 0.89 pad 1.65)
  other vias: 25.4,29.84
N$186  (via drill 0.89 pad 1.65)
  other vias: 27.94,29.84
N$187  (via drill 0.89 pad 1.65)
  other vias: 45.72,27.3
N$188  (via drill 0.89 pad 1.65)
  other vias: 30.48,29.84
N$189  (via drill 0.89 pad 1.65)
  other vias: 33.02,29.84
N$190  (via drill 0.89 pad 1.65)
  other vias: 10.16,32.38
N$191  (via drill 0.89 pad 1.65)
  other vias: 12.7,32.38
N$192  (via drill 0.89 pad 1.65)
  other vias: 15.24,32.38
N$193  (via drill 0.89 pad 1.65)
  other vias: 17.78,32.38
N$194  (via drill 0.89 pad 1.65)
  other vias: 20.32,32.38
N$195  (via drill 0.89 pad 1.65)
  other vias: 22.86,32.38
N$196  (via drill 0.89 pad 1.65)
  other vias: 25.4,32.38
N$197  (via drill 0.89 pad 1.65)
  other vias: 27.94,32.38
N$198  (via drill 0.89 pad 1.65)
  other vias: 30.48,32.38
N$199  (via drill 0.89 pad 1.65)
  other vias: 33.02,32.38
N$200  (via drill 0.89 pad 1.65)
  other vias: 12.7,34.92
N$201  (via drill 0.89 pad 1.65)
  other vias: 15.24,34.92
N$202  (via drill 0.89 pad 1.65)
  other vias: 17.78,34.92
N$203  (via drill 0.89 pad 1.65)
  other vias: 20.32,34.92
N$204  (via drill 0.89 pad 1.65)
  other vias: 22.86,34.92
N$205  (via drill 0.89 pad 1.65)
  other vias: 25.4,34.92
N$206  (via drill 0.89 pad 1.65)
  other vias: 27.94,34.92
N$207  (via drill 0.89 pad 1.65)
  other vias: 30.48,34.92
N$208  (via drill 0.89 pad 1.65)
  other vias: 33.02,34.92
N$209  (via drill 0.89 pad 1.65)
  other vias: 35.56,34.92
N$210  (via drill 0.89 pad 1.65)
  other vias: 35.56,32.38
N$211  (via drill 0.89 pad 1.65)
  other vias: 35.56,29.84
N$212  (via drill 0.89 pad 1.65)
  other vias: 35.56,27.3
N$213  (via drill 0.89 pad 1.65)
  other vias: 35.56,24.77
N$214  (via drill 0.89 pad 1.65)
  other vias: 55.88,6.99
N$215  (via drill 0.89 pad 1.65)
  other vias: 35.56,17.14
N$216  (via drill 0.89 pad 1.65)
  other vias: 7.62,29.84
N$217  (via drill 0.89 pad 1.65)
  other vias: 55.88,4.45
N$218  (via drill 0.89 pad 1.65)
  other vias: 35.56,14.61
N$219  (via drill 0.89 pad 1.65)
  other vias: 7.62,32.38
N$220  (via drill 0.89 pad 1.65)
  other vias: 33.02,22.23
N$221  (via drill 0.89 pad 1.65)
  other vias: 7.62,34.92
N$222  (via drill 0.89 pad 1.65)
  other vias: 38.1,37.47
N$223  (via drill 0.89 pad 1.65)
  other vias: 40.64,37.47
N$224  (via drill 0.89 pad 1.65)
  other vias: 43.18,37.47
N$225  (via drill 0.89 pad 1.65)
  other vias: 45.72,37.47
N$226  (via drill 0.89 pad 1.65)
  other vias: 48.26,37.47
N$227  (via drill 0.89 pad 1.65)
  other vias: 50.8,37.47
N$228  (via drill 0.89 pad 1.65)
  other vias: 53.34,37.47
N$229  (via drill 0.89 pad 1.65)
  other vias: 55.88,37.47
N$230  (via drill 0.89 pad 1.65)
  other vias: 58.42,37.47
N$231  (via drill 0.89 pad 1.65)
  other vias: 48.26,27.3
N$232  (via drill 0.89 pad 1.65)
  other vias: 60.96,37.47
N$233  (via drill 0.89 pad 1.65)
  other vias: 40.64,40.01
N$234  (via drill 0.89 pad 1.65)
  other vias: 43.18,40.01
N$235  (via drill 0.89 pad 1.65)
  other vias: 45.72,40.01
N$236  (via drill 0.89 pad 1.65)
  other vias: 48.26,40.01
N$237  (via drill 0.89 pad 1.65)
  other vias: 50.8,40.01
N$238  (via drill 0.89 pad 1.65)
  other vias: 53.34,40.01
N$239  (via drill 0.89 pad 1.65)
  other vias: 55.88,40.01
N$240  (via drill 0.89 pad 1.65)
  other vias: 58.42,40.01
N$241  (via drill 0.89 pad 1.65)
  other vias: 60.96,40.01
N$242  (via drill 0.89 pad 1.65)
  other vias: 63.5,40.01
N$243  (via drill 0.89 pad 1.65)
  other vias: 63.5,37.47
N$244  (via drill 0.89 pad 1.65)
  other vias: 10.16,37.47
N$245  (via drill 0.89 pad 1.65)
  other vias: 12.7,37.47
N$246  (via drill 0.89 pad 1.65)
  other vias: 15.24,37.47
N$247  (via drill 0.89 pad 1.65)
  other vias: 17.78,37.47
N$248  (via drill 0.89 pad 1.65)
  other vias: 20.32,37.47
N$249  (via drill 0.89 pad 1.65)
  other vias: 22.86,37.47
N$250  (via drill 0.89 pad 1.65)
  other vias: 25.4,37.47
N$251  (via drill 0.89 pad 1.65)
  other vias: 27.94,37.47
N$252  (via drill 0.89 pad 1.65)
  other vias: 30.48,37.47
N$253  (via drill 0.89 pad 1.65)
  other vias: 33.02,37.47
N$254  (via drill 0.89 pad 1.65)
  other vias: 12.7,40.01
N$255  (via drill 0.89 pad 1.65)
  other vias: 15.24,40.01
N$256  (via drill 0.89 pad 1.65)
  other vias: 17.78,40.01
N$257  (via drill 0.89 pad 1.65)
  other vias: 20.32,40.01
N$258  (via drill 0.89 pad 1.65)
  other vias: 22.86,40.01
N$259  (via drill 0.89 pad 1.65)
  other vias: 25.4,40.01
N$260  (via drill 0.89 pad 1.65)
  other vias: 27.94,40.01
N$261  (via drill 0.89 pad 1.65)
  other vias: 30.48,40.01
N$262  (via drill 0.89 pad 1.65)
  other vias: 33.02,40.01
N$263  (via drill 0.89 pad 1.65)
  other vias: 35.56,40.01
N$264  (via drill 0.89 pad 1.65)
  other vias: 35.56,37.47
N$265  (via drill 0.89 pad 1.65)
  other vias: 7.62,24.77
N$266  (via drill 0.89 pad 1.65)
  other vias: 7.62,22.23
N$267  (via drill 0.89 pad 1.65)
  other vias: 7.62,37.47
N$268  (via drill 0.89 pad 1.65)
  other vias: 33.02,14.61
N$269  (via drill 0.89 pad 1.65)
  other vias: 7.62,40.01
N$271  (via drill 0.89 pad 1.65)
  other vias: 30.48,22.23
N$275  (via drill 0.89 pad 1.65)
  other vias: 50.8,27.3
N$278  (via drill 0.89 pad 1.65)
  other vias: 12.7,12.06
N$279  (via drill 0.89 pad 1.65)
  other vias: 12.7,9.53
N$280  (via drill 0.89 pad 1.65)
  other vias: 38.1,34.92
N$281  (via drill 0.89 pad 1.65)
  other vias: 15.24,12.06
N$282  (via drill 0.89 pad 1.65)
  other vias: 15.24,9.53
N$283  (via drill 0.89 pad 1.65)
  other vias: 17.78,12.06
N$284  (via drill 0.89 pad 1.65)
  other vias: 17.78,9.53
N$286  (via drill 0.89 pad 1.65)
  other vias: 20.32,12.06
N$287  (via drill 0.89 pad 1.65)
  other vias: 20.32,9.53
N$288  (via drill 0.89 pad 1.65)
  other vias: 22.86,12.06
N$289  (via drill 0.89 pad 1.65)
  other vias: 22.86,9.53
N$290  (via drill 0.89 pad 1.65)
  other vias: 25.4,12.06
N$291  (via drill 0.89 pad 1.65)
  other vias: 25.4,9.53
N$292  (via drill 0.89 pad 1.65)
  other vias: 27.94,12.06
N$293  (via drill 0.89 pad 1.65)
  other vias: 27.94,9.53
N$294  (via drill 0.89 pad 1.65)
  other vias: 30.48,12.06
N$295  (via drill 0.89 pad 1.65)
  other vias: 30.48,9.53
N$296  (via drill 0.89 pad 1.65)
  other vias: 33.02,12.06
N$297  (via drill 0.89 pad 1.65)
  other vias: 33.02,9.53
N$298  (via drill 0.89 pad 1.65)
  other vias: 12.7,14.61
N$299  (via drill 0.89 pad 1.65)
  other vias: 15.24,14.61
N$300  (via drill 0.89 pad 1.65)
  other vias: 17.78,14.61
N$301  (via drill 0.89 pad 1.65)
  other vias: 20.32,14.61
N$302  (via drill 0.89 pad 1.65)
  other vias: 22.86,14.61
N$303  (via drill 0.89 pad 1.65)
  other vias: 25.4,14.61
N$304  (via drill 0.89 pad 1.65)
  other vias: 35.56,12.06
N$305  (via drill 0.89 pad 1.65)
  other vias: 12.7,17.14
N$306  (via drill 0.89 pad 1.65)
  other vias: 15.24,17.14
N$307  (via drill 0.89 pad 1.65)
  other vias: 17.78,17.14
N$308  (via drill 0.89 pad 1.65)
  other vias: 20.32,17.14
N$309  (via drill 0.89 pad 1.65)
  other vias: 22.86,17.14
N$310  (via drill 0.89 pad 1.65)
  other vias: 25.4,17.14
N$311  (via drill 0.89 pad 1.65)
  other vias: 35.56,9.53
N$312  (via drill 0.89 pad 1.65)
  other vias: 12.7,6.99
N$313  (via drill 0.89 pad 1.65)
  other vias: 12.7,4.45
N$314  (via drill 0.89 pad 1.65)
  other vias: 15.24,6.99
N$315  (via drill 0.89 pad 1.65)
  other vias: 15.24,4.45
N$316  (via drill 0.89 pad 1.65)
  other vias: 17.78,6.99
N$317  (via drill 0.89 pad 1.65)
  other vias: 17.78,4.45
N$318  (via drill 0.89 pad 1.65)
  other vias: 20.32,6.99
N$319  (via drill 0.89 pad 1.65)
  other vias: 53.34,27.3
N$320
  Top 0.305: R1.1 LED_A.1
N$321  (via drill 0.89 pad 1.65)
  other vias: 20.32,4.45
N$322  (via drill 0.89 pad 1.65)
  other vias: 22.86,6.99
N$323  (via drill 0.89 pad 1.65)
  other vias: 22.86,4.45
N$324  (via drill 0.89 pad 1.65)
  other vias: 25.4,6.99
N$325  (via drill 0.89 pad 1.65)
  other vias: 25.4,4.45
N$326  (via drill 0.89 pad 1.65)
  other vias: 27.94,6.99
N$327  (via drill 0.89 pad 1.65)
  other vias: 27.94,4.45
N$328  (via drill 0.89 pad 1.65)
  other vias: 30.48,1.91
N$329  (via drill 0.89 pad 1.65)
  other vias: 33.02,1.91
N$330  (via drill 0.89 pad 1.65)
  other vias: 12.7,19.68
N$331  (via drill 0.89 pad 1.65)
  other vias: 15.24,19.68
N$332  (via drill 0.89 pad 1.65)
  other vias: 17.78,19.68
N$333  (via drill 0.89 pad 1.65)
  other vias: 20.32,19.68
N$334  (via drill 0.89 pad 1.65)
  other vias: 22.86,19.68
N$335  (via drill 0.89 pad 1.65)
  other vias: 25.4,19.68
N$336
  Top 0.305: R15.1 81.03,30.35 Q4.3 81.03,26.92 80.14,26.04 73.09,26.04 72.14,26.99 C1.1
N$337  (via drill 0.89 pad 1.65)
  other vias: 12.7,22.23
N$338  (via drill 0.89 pad 1.65)
  other vias: 15.24,22.23
N$339  (via drill 0.89 pad 1.65)
  other vias: 17.78,22.23
N$340  (via drill 0.89 pad 1.65)
  other vias: 20.32,22.23
N$341  (via drill 0.89 pad 1.65)
  other vias: 22.86,22.23
N$342  (via drill 0.89 pad 1.65)
  other vias: 25.4,22.23
N$343  (via drill 0.89 pad 1.65)
  other vias: 35.56,1.91
N$344  (via drill 0.89 pad 1.65)
  other vias: 38.1,1.91
N$345  (via drill 0.89 pad 1.65)
  other vias: 40.64,1.91
N$346  (via drill 0.89 pad 1.65)
  other vias: 43.18,1.91
N$347
  Top 0.305: R2.2 78.99,49.4 Q7.1 R3.1 R4.1
N$348  (via drill 0.89 pad 1.65)
  other vias: 30.48,14.61
N$349  (via drill 0.89 pad 1.65)
  other vias: 45.72,1.91
N$350  (via drill 0.89 pad 1.65)
  other vias: 48.26,1.91
N$351  (via drill 0.89 pad 1.65)
  other vias: 50.8,1.91
N$352  (via drill 0.89 pad 1.65)
  other vias: 53.34,1.91
N$353  (via drill 0.89 pad 1.65)
  other vias: 55.88,1.91
N$354  (via drill 0.89 pad 1.65)
  other vias: 12.7,1.91
N$359  (via drill 0.89 pad 1.65)
  other vias: 15.24,1.91
N$360  (via drill 0.89 pad 1.65)
  other vias: 17.78,1.91
N$361  (via drill 0.89 pad 1.65)
  other vias: 20.32,1.91
N$362  (via drill 0.89 pad 1.65)
  other vias: 22.86,1.91
N$363  (via drill 0.89 pad 1.65)
  other vias: 55.88,27.3
N$364  (via drill 0.89 pad 1.65)
  other vias: 25.4,1.91
N$365  (via drill 0.89 pad 1.65)
  other vias: 27.94,1.91
N$366  (via drill 0.89 pad 1.65)
  other vias: 27.94,22.23
N$367  (via drill 0.89 pad 1.65)
  other vias: 27.94,19.68
N$368  (via drill 0.89 pad 1.65)
  other vias: 27.94,17.14
N$369  (via drill 0.89 pad 1.65)
  other vias: 27.94,14.61
N$370
  Top 0.61: S.1 R3.2 R5.2
N$373
  Top 0.61: Q1.2 R6.1 76.96,38.99 76.45,38.48 73.28,38.48 72.01,39.75 D1.1
N$374
  Top 0.305: R4.2 G.1
N$375
  Top 0.61: R5.1 Q7.2
N$376
  Top 0.305: Q1.1 77.09,41.53 | 77.09,41.53 R7.1 R8.1 | R6.2 75.44,39.88 77.09,41.53
N$377
  Top 0.406: R9.1 PWR.+
N$378
  Top 0.305: R15.2 78.99,30.35 Q4.1 R16.1 R17.1
N$379
  Top 0.305: R18.2 R16.2 E1.1
N$380
  Top 0.305: R17.2 B1.1
N$381
  Top 0.305: Q4.2 R18.1
N$383  (via drill 0.3 pad 0.64)
  Top 0.61: S1.1 v74.55,41.53 R7.2 | R10.2 v78.36,43.43
  Bottom 0.61: v78.36,43.43 76.45,43.43 v74.55,41.53
N$384
  Top 0.305: R8.2 G1.1
N$385
  Top 0.61: D.1 72.14,46.1 73.53,44.7 80.01,44.7 81.03,45.72 Q7.3 81.03,49.4 R2.1
N$386
  Top 0.305: Q2.2 R11.1 76.96,33.27 76.07,32.38 73.15,32.38 72.14,33.4 E.1
N$387
  Top 0.305: Q2.1 R12.1 | R12.1 R13.1 | R11.2 75.44,33.53 76.71,34.8 76.71,34.92 R12.1
N$388  (via drill 0.3 pad 0.64)
  Top 0.305: R12.2 v74.55,35.18 C.1 | R14.2 v78.36,36.96
  Bottom 0.305: v78.36,36.96 76.33,36.96 v74.55,35.18
N$389
  Top 0.305: A.1 D5.+
N$390
  Top 0.305: K.1 79.88,17.78 82.17,15.49 D5.-
N$391
  Top 0.305: LED1.+ R1.2
N$392
  Top 0.305: LED_K.1 78.23,22.86 LED1.-
N$393
  Top 0.305: TP5.1 K1.1 K1.4
N$394
  Top 0.305: TP6.1 K1.2 K1.3
N$395
  Top 0.61: Q1.3 81.03,43.18 R10.1
N$396
  Top 0.305: B.1 R13.2
N$397
  Top 0.305: Q2.3 81.03,36.7 R14.1
N$407  (via drill 0.89 pad 1.65)
  other vias: 58.42,27.3
N$451  (via drill 0.89 pad 1.65)
  other vias: 60.96,27.3

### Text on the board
tPlace: B+ | 5V | 5V | B+ | GND | TXD | RXD | GP18 | GND | GP23 | GP24 | GND | GP25 | CS0 | CS1 | SC | GND | GP12 | GND | GP16 | GP20 | GP21 | P-MOS | 3V3 | GP2 | GP3 | GP4 | GND | GP17 | GP27 | GP22 | 3V3 | MOSI | MISO | SCLK | GND | SD | GP5 | GP6 | GP13 | GP19 | GP26 | GND | B | N-MOS | NPN | PNP | B | 5V | D- | D+ | GND | B+ | B+
bPlace: www.seeedstudio.com | by Seeed Studio | v1.0 11/10/2014 | Raspberry Pi Breakout Board

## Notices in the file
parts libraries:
moudle-new: This work is licensed under the Creative Commons Attribution 4.0 International License.
To view a copy of this license,visit:
http://creativecommons.org/licenses/by-sa/4.0
moudle-new: CC-BY-SA
